[IBIS Ver]   3.2
[File name]   sprm160.ibs
[File Rev]   1.1
[Date]   Tue Mar 4 14:22:13 US/Central 2003
[Source]   IBIS Model Generated from PACED 4.51D
|   Technology type SR40
[Disclaimer]   Please be aware that in the absence of a written agreement
|   Texas Instruments(TI) assumes no liability for:
|   (1) The accuracy of the IBIS models provided to your company
|   (2) The proper functioning of these Models in your design
|   or for any resulting applications;or
|   property rights resulting from your use of these models.
|   TI provides IBIS Models as a service to our customers and
|   therefore reserves the right to limit distribution of the
|   Models.
[Copyright]   Property of Texas Instruments Incorporated.
|   Unauthorised reproduction and/or distribution is strictly.
|   prohibited.
|   This product is protected under copyright law and trade
|   secret law as an unpublished work.
|   Created 1999,(C) Copyright 1999-2001,
|   Texas Instruments Incorporated., All Rights Reserved.
[Notes]
|   File Rev 1.0:   Original
|   File Rev 1.1:   Corrected EMIF address pin names.
|   Corrected EMIF clock pin names.
|   Removed PLLSENSE pin, this pin is NC pin.
[Component]   TMS320VC5501_PGF   | 176 pin
[Manufacturer]   Texas Instruments
[Package]
| Variable   Typ   Min   Max
R_pkg   0.2266   0.2072   0.2485
L_pkg   8.426e-09   7.749e-09   9.656e-09
C_pkg   2.053e-12   1.825e-12   2.396e-12
[Pin]   signal_name   model_name   R_pin   L_pin   C_pin
1   GPIO6   idi041_ouk831   0.2104   9.651e-09   1.879e-12
2   GPIO4   idi041_ouk831   0.2120   9.320e-09   2.383e-12
3   GPIO2   idi041_ouk831   0.2139   9.142e-09   2.341e-12
4   GPIO1   idi041_ouk831   0.2160   9.007e-09   2.297e-12
5   GPIO0   idi041_ouk831   0.2183   8.891e-09   2.253e-12
6   TIM1   idi041_ouk831   0.2207   8.786e-09   2.209e-12
7   TIM0   idi041_ouk831   0.2233   8.692e-09   2.166e-12
8   NINT0   idg091   0.2261   8.607e-09   2.124e-12
9   POWER   NC   0.2288   8.532e-09   2.085e-12
10   NINT1   idg091   0.2334   8.497e-09   2.095e-12
11   NINT2   idg091   0.2365   8.491e-09   2.139e-12
12   POWER   NC   0.2371   8.415e-09   2.107e-12
13   NINT3   idg091   0.2380   8.278e-09   2.000e-12
14   NNMI   idg091_ouk831_ps1001   0.2380   8.193e-09   1.929e-12
15   NIACK   ouk831   0.2391   8.127e-09   1.910e-12
16   GND   NC   0.2404   8.074e-09   1.893e-12
17   CLKR0   idg091_ouk831   0.2408   8.032e-09   1.878e-12
18   DR0   idg041   0.2423   8.001e-09   1.864e-12
19   FSR0   idi041_ouk831   0.2439   7.985e-09   1.853e-12
20   CLKX0   idg091_ouk831   0.2456   7.995e-09   1.846e-12
21   POWER   NC   0.2465   7.974e-09   1.901e-12
22   DX0   ouk831   0.2482   8.112e-09   2.010e-12
23   FSX0   idi041_ouk831   0.2485   8.110e-09   2.011e-12
24   CLKR1   idg091_ouk831   0.2471   7.972e-09   1.900e-12
25   DR1   idg041   0.2458   7.956e-09   1.829e-12
26   FSR1   idi041_ouk831   0.2450   7.966e-09   1.843e-12
27   DX1   ouk831   0.2438   8.017e-09   1.865e-12
28   CLKX1   idg091_ouk831   0.2428   8.055e-09   1.880e-12
29   GND   NC   0.2419   8.092e-09   1.897e-12
30   FSX1   idi041_ouk831   0.2410   8.150e-09   1.916e-12
31   TEST01   idg041   0.2402   8.221e-09   1.937e-12
32   NC02   ouk831   0.2405   8.312e-09   2.009e-12
33   POWER   NC   0.2385   8.436e-09   2.109e-12
34   RX   idi041_ouk831   0.2367   8.495e-09   2.137e-12
35   GPIO5   idi041_ouk831   0.2337   8.500e-09   2.101e-12
36   POWER   NC   0.2308   8.556e-09   2.091e-12
37   TX   idg091_ouk831   0.2281   8.633e-09   2.132e-12
38   GPIO3   idg091_ouk831   0.2255   8.720e-09   2.175e-12
39   GND   NC   0.2231   8.818e-09   2.219e-12
40   SCL   idi091_uos205   0.2208   8.925e-09   2.264e-12
41   SDA   idi091_uos205   0.2188   9.047e-09   2.309e-12
42   HC1   idg091_ouk831_pe1001   0.2143   9.152e-09   2.354e-12
43   HC0   idg091_ouk831_ps1001   0.2125   9.333e-09   2.396e-12
44   NHCS   idg091_ouk831_ps1001   0.2108   9.656e-09   1.887e-12
45   HCNTL1   idi041_ouk831_ps1001   0.2072   9.613e-09   1.878e-12
46   HCNTL0   idi041_ouk831_ps1001   0.2077   9.267e-09   2.382e-12
47   GND   NC   0.2084   9.075e-09   2.340e-12
48   HRNW   idi041_ouk831_ps1001   0.2094   8.927e-09   2.295e-12
49   NHDS2   idg091_ouk831_ps1001   0.2107   8.798e-09   2.250e-12
50   POWER   NC   0.2123   8.682e-09   2.205e-12
51   NHDS1   idg091_ouk831_ps1001   0.2163   8.605e-09   2.163e-12
52   HRDY   idi041_ouk831_ps1001   0.2181   8.509e-09   2.121e-12
53   POWER   NC   0.2201   8.425e-09   2.080e-12
54   CLKOUT   oukb31   0.2223   8.360e-09   2.091e-12
55   XF   ouk831   0.2250   8.349e-09   2.135e-12
56   GND   NC   0.2250   8.265e-09   2.104e-12
57   C15   ups312_ouk831   0.2253   8.121e-09   1.997e-12
58   C14   idi041_ouk831_ps1001   0.2247   8.029e-09   1.925e-12
59   NHINT   idi041_ouk831_ps1001   0.2253   7.957e-09   1.906e-12
60   POWER   NC   0.2261   7.898e-09   1.889e-12
61   NC01   NC   0.2261   7.851e-09   1.873e-12
62   X1   NC   0.2272   7.814e-09   1.860e-12
63   X2CLKIN   NC   0.2285   7.794e-09   1.848e-12
64   EMIFCLKS   idg091   0.2299   7.801e-09   1.841e-12
65   GND   NC   0.2305   7.776e-09   1.896e-12
66   C13   ups312_ouk831   0.2322   7.914e-09   2.005e-12
67   C12   ups312_ouk831   0.2322   7.909e-09   2.006e-12
68   C11   ups312_ouk831   0.2307   7.769e-09   1.895e-12
69   C10   ups312_ouk831   0.2292   7.751e-09   1.825e-12
70   C9   ups312_ouk831   0.2290   7.768e-09   1.839e-12
71   C8   ups312_ouk831   0.2278   7.819e-09   1.861e-12
72   C7   ups312_ouk831   0.2269   7.859e-09   1.876e-12
73   GND   NC   0.2271   7.909e-09   1.893e-12
74   ECLKIN   NC   0.2265   7.971e-09   1.912e-12
75   ECLKOUT2   ouk831   0.2260   8.046e-09   1.933e-12
76   ECLKOUT1   ouk831   0.2267   8.142e-09   2.004e-12
77   POWER   NC   0.2250   8.269e-09   2.102e-12
78   C6   ups312_ouk831   0.2234   8.330e-09   2.132e-12
79   C5   ups312_ouk831   0.2208   8.342e-09   2.097e-12
80   POWER   NC   0.2185   8.405e-09   2.088e-12
81   C4   ups312_ouk831   0.2163   8.489e-09   2.129e-12
82   C3   idi041_ouk831_ps1001   0.2144   8.584e-09   2.172e-12
83   GND   NC   0.2127   8.690e-09   2.216e-12
84   C2   ups312_ouk831   0.2112   8.807e-09   2.261e-12
85   C1   ups312_ouk831   0.2099   8.938e-09   2.307e-12
86   C0   ups312_ouk831   0.2089   9.087e-09   2.353e-12
87   A21   ups312_ouk831   0.2082   9.281e-09   2.395e-12
88   A20   ups312_ouk831   0.2078   9.620e-09   1.887e-12
89   A19   ups312_ouk831   0.2104   9.651e-09   1.879e-12
90   A18   ups312_ouk831   0.2121   9.321e-09   2.383e-12
91   GND   NC   0.2140   9.144e-09   2.342e-12
92   A17   ups312_ouk831   0.2161   9.009e-09   2.297e-12
93   A16   ups312_ouk831   0.2184   8.893e-09   2.253e-12
94   POWER   NC   0.2209   8.788e-09   2.209e-12
95   A15   ups312_ouk831   0.2236   8.694e-09   2.166e-12
96   A14   ups312_ouk831   0.2263   8.610e-09   2.124e-12
97   GND   NC   0.2293   8.537e-09   2.083e-12
98   A13   ups312_ouk831   0.2323   8.483e-09   2.094e-12
99   A12   ups312_ouk831   0.2355   8.479e-09   2.138e-12
100   POWER   NC   0.2374   8.419e-09   2.109e-12
101   A11   ups312_ouk831   0.2394   8.295e-09   2.001e-12
102   A10   ups312_ouk831   0.2392   8.208e-09   1.929e-12
103   A9   ups312_ouk831   0.2402   8.140e-09   1.910e-12
104   A8   ups312_ouk831   0.2412   8.085e-09   1.894e-12
105   POWER   NC   0.2414   8.040e-09   1.878e-12
106   A7   ups312_ouk831   0.2428   8.007e-09   1.864e-12
107   A6   ups312_ouk831   0.2442   7.988e-09   1.853e-12
108   A5   ups312_ouk831   0.2457   7.997e-09   1.846e-12
109   GND   NC   0.2464   7.973e-09   1.901e-12
110   A4   ups312_ouk831   0.2481   8.111e-09   2.009e-12
111   A3   ups312_ouk831   0.2482   8.106e-09   2.011e-12
112   A2   ups312_ouk831   0.2465   7.966e-09   1.900e-12
113   POWER   NC   0.2451   7.947e-09   1.829e-12
114   D31   ups312_ouk831   0.2447   7.963e-09   1.844e-12
115   D30   ups312_ouk831   0.2434   8.012e-09   1.865e-12
116   D29   ups312_ouk831   0.2423   8.049e-09   1.879e-12
117   GND   NC   0.2414   8.085e-09   1.897e-12
118   D28   ups312_ouk831   0.2403   8.142e-09   1.916e-12
119   D27   ups312_ouk831   0.2394   8.212e-09   1.937e-12
120   D26   ups312_ouk831   0.2396   8.300e-09   2.008e-12
121   POWER   NC   0.2375   8.424e-09   2.109e-12
122   D25   ups312_ouk831   0.2357   8.482e-09   2.137e-12
123   D24   ups312_ouk831   0.2325   8.486e-09   2.100e-12
124   POWER   NC   0.2295   8.540e-09   2.091e-12
125   D23   ups312_ouk831   0.2266   8.615e-09   2.132e-12
126   D22   ups312_ouk831   0.2238   8.700e-09   2.175e-12
127   D21   ups312_ouk831   0.2213   8.795e-09   2.219e-12
128   D20   ups312_ouk831   0.2188   8.900e-09   2.263e-12
129   D19   ups312_ouk831   0.2165   9.019e-09   2.309e-12
130   GND   NC   0.2144   9.154e-09   2.355e-12
131   D18   ups312_ouk831   0.2125   9.333e-09   2.396e-12
132   D17   ups312_ouk831   0.2108   9.656e-09   1.887e-12
133   D16   ups312_ouk831   0.2072   9.613e-09   1.878e-12
134   D15   ups312_ouk831   0.2078   9.268e-09   2.382e-12
135   D14   ups312_ouk831   0.2086   9.077e-09   2.340e-12
136   D13   ups312_ouk831   0.2097   8.930e-09   2.295e-12
137   D12   ups312_ouk831   0.2110   8.801e-09   2.250e-12
138   D11   ups312_ouk831   0.2126   8.686e-09   2.205e-12
139   D10   ups312_ouk831   0.2167   8.610e-09   2.163e-12
140   D9   ups312_ouk831   0.2186   8.514e-09   2.121e-12
141   POWER   NC   0.2206   8.430e-09   2.080e-12
142   D8   ups312_ouk831   0.2228   8.366e-09   2.091e-12
143   D7   ups312_ouk831   0.2252   8.352e-09   2.135e-12
144   GND   NC   0.2252   8.268e-09   2.104e-12
145   D6   ups312_ouk831   0.2255   8.123e-09   1.997e-12
146   D5   ups312_ouk831   0.2249   8.032e-09   1.925e-12
147   D4   ups312_ouk831   0.2256   7.960e-09   1.906e-12
148   POWER   NC   0.2263   7.901e-09   1.888e-12
149   D3   ups312_ouk831   0.2271   7.864e-09   1.873e-12
150   D2   ups312_ouk831   0.2281   7.825e-09   1.860e-12
151   D1   ups312_ouk831   0.2292   7.802e-09   1.848e-12
152   D0   ups312_ouk831   0.2304   7.807e-09   1.842e-12
153   GND   NC   0.2308   7.780e-09   1.897e-12
154   EMU1   NC   0.2323   7.914e-09   2.006e-12
155   EMU0   NC   0.2322   7.909e-09   2.007e-12
156   TDO   ouk831   0.2305   7.768e-09   1.895e-12
157   GND   NC   0.2291   7.749e-09   1.825e-12
158   TDI   idi041_ps1001   0.2287   7.765e-09   1.839e-12
159   TRSTN   idg091_pe1001   0.2275   7.815e-09   1.861e-12
160   TCK   idi091_ps1001   0.2264   7.853e-09   1.876e-12
161   TMS   idi041_ps1001   0.2265   7.902e-09   1.893e-12
162   NRESET   NC   0.2258   7.962e-09   1.912e-12
163   HPIENA   NC   0.2252   8.036e-09   1.933e-12
164   HD7   ups312_ouk831   0.2257   8.130e-09   2.005e-12
165   POWER   NC   0.2253   8.274e-09   2.106e-12
166   HD6   ups312_ouk831   0.2238   8.335e-09   2.133e-12
167   HD5   ups312_ouk831   0.2213   8.347e-09   2.097e-12
168   POWER   NC   0.2189   8.410e-09   2.088e-12
169   HD4   ups312_ouk831   0.2167   8.494e-09   2.129e-12
170   HD3   ups312_ouk831   0.2148   8.588e-09   2.172e-12
171   POWER   NC   0.2130   8.694e-09   2.216e-12
172   HD2   ups312_ouk831   0.2115   8.810e-09   2.262e-12
173   HD1   ups312_ouk831   0.2102   8.941e-09   2.307e-12
174   GND   NC   0.2091   9.089e-09   2.353e-12
175   HD0   ups312_ouk831   0.2083   9.282e-09   2.395e-12
176   GPIO7   NC   0.2079   9.620e-09   1.886e-12
| Models and submodels in the file (14): idg041 (Input), idg091 (Input), ouk831 (3-state), oukb31 (3-state), idg091_ouk831 (I/O), idg091_ouk831_ps1001 (I/O), idg091_pe1001 (Input), idi041_ouk831 (I/O), idi041_ouk831_ps1001 (I/O), idi041_ps1001 (Input), idi091_ps1001 (Input), idi091_uos205 (I/O_open_drain), ups312_ouk831 (I/O), idg091_ouk831_pe1001 (I/O)
